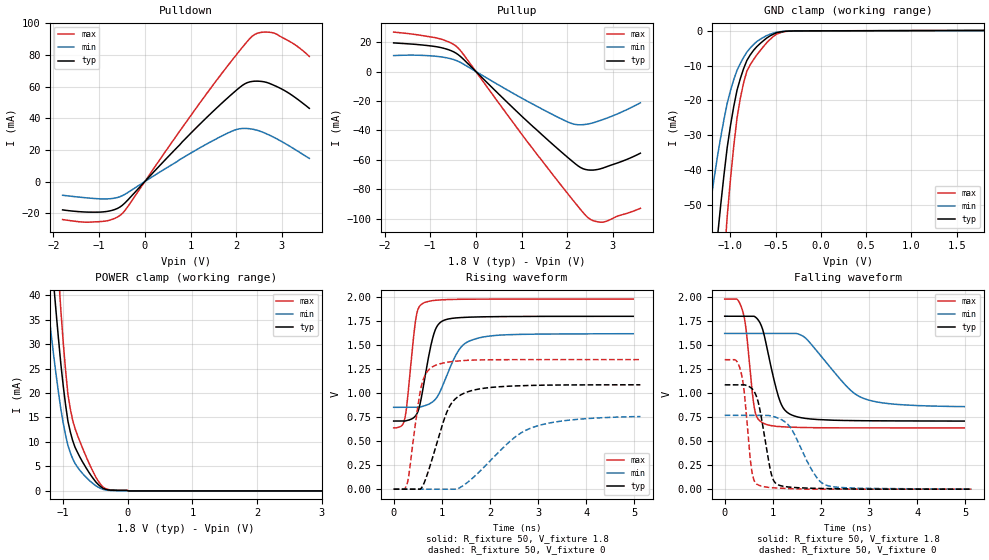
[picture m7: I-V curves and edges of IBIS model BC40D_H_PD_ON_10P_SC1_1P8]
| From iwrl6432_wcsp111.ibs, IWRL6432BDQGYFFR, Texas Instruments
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|   Model Cell BC40D_H_PD_ON_10P_SC1_1P8
|BC40D_H_PD_ON_10P_SC1_1P8
[Model]   BC40D_H_PD_ON_10P_SC1_1P8
Model_type   I/O
Polarity   Non-Inverting
Enable   Active-Low
Vinl =  0.63
Vinh =  1.17
Cref =  15pF
Rref =  100.0000M
Vref =  0V
Vmeas =  0.9
C_comp   2.389419p   2.292106p   2.408415p
|[Input load] weak_pd_on
|[Output drive] slow
|[supplytol] 10
|[temp] ind
[Model Spec]
Vinl   0.63   0.567   0.693
Vinh   1.17   1.053   1.287
[Temperature Range]   25   125   -40
[Voltage Range]   1.8   1.62   1.98
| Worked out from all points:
|   slope of the pulldown table from 0 to 0.27 V, typ, clamps not added: 32.2 ohm
|   slope of the pullup table from 0 to 0.27 V, typ, clamps not added: 32.6 ohm
|   GND clamp passes 1 mA (typ) near -0.53 V on its own axis
|   POWER clamp passes 1 mA (typ) near -0.43 V on its own axis
|   rising waveform, R_fixture 50, V_fixture 1.8: 20-80 % time 249ps typ, 424ps min, 162ps max; typ from 0.709 V to 1.8 V
|   rising waveform, R_fixture 50, V_fixture 0: 20-80 % time 429ps typ, 994ps min, 231ps max; typ from 0 V to 1.09 V
|   falling waveform, R_fixture 50, V_fixture 1.8: 20-80 % time 310ps typ, 792ps min, 166ps max; typ from 1.8 V to 0.708 V
|   falling waveform, R_fixture 50, V_fixture 0: 20-80 % time 227ps typ, 467ps min, 151ps max; typ from 1.08 V to 0 V
| Nom Voltages:
|   VDD=1.1001, VDDS=1.8, VDDS18=1.8, ESD_BIASFET=0, VSS=0, VSSS=0
| Min Voltages:
|   VDD=0.99, VDDS=1.62, VDDS18=1.62, ESD_BIASFET=0, VSS=0, VSSS=0
| Max Voltages:
|   VDD=1.21, VDDS=1.98, VDDS18=1.98, ESD_BIASFET=0, VSS=0, VSSS=0
[POWER_clamp]
|   voltage   I(typ)   I(min)   I(max)
-1.8V     158.9mA    112.6mA    219.9mA
-1.255V   60.04mA    40.04mA    85.04mA
-1.145V   41.99mA    27.45mA    59.9mA
-1.109V   36.4mA     23.66mA    51.96mA
-1.073V   31.03mA    20.08mA    44.3mA
-1.036V   25.91mA    16.71mA    36.9mA
-927.3mV  14.27mA    9.297mA    19.77mA
-854.5mV  10.33mA    6.619mA    14.49mA
-454.5mV  1.273mA    741.7uA    1.94mA
-309.1mV  221.6uA    132.8uA    307.9uA
18.18mV   0A         0A         0A
3.6V      0A         0A         0A
[Pulldown]
|   voltage   I(typ)   I(min)   I(max)
-1.8V     -17.92mA   -8.674mA   -24.03mA
-927.3mV  -19.22mA   -10.99mA   -25.2mA
-654.5mV  -17.65mA   -10.46mA   -23.22mA
-490.9mV  -14.97mA   -8.904mA   -20.12mA
818.2mV   25.05mA    14.78mA    34.16mA
1.691V    49.7mA     28.87mA    68.58mA
2.127V    60.63mA    33.53mA    84.59mA
2.4V      63.43mA    32.85mA    92.9mA
2.618V    62.99mA    30.74mA    94.47mA
2.836V    60.69mA    27.76mA    93.76mA
3.273V    53.49mA    20.53mA    86.73mA
3.6V      46.26mA    14.64mA    79.12mA
[Pullup]
|   voltage   I(typ)   I(min)   I(max)
-1.8V     19.42mA    10.82mA    26.76mA
-818.2mV  16.58mA    10.15mA    22.47mA
-545.5mV  14.19mA    8.648mA    19.37mA
-381.8mV  11.34mA    6.842mA    15.75mA
1.036V    -31.26mA   -18.6mA    -43.9mA
1.909V    -55.59mA   -32.73mA   -78.89mA
2.182V    -62.71mA   -35.92mA   -89.46mA
2.345V    -65.94mA   -36.05mA   -95.62mA
2.455V    -66.75mA   -35.58mA   -99.18mA
2.618V    -66.67mA   -34.29mA   -101.7mA
2.782V    -65.46mA   -32.56mA   -102.2mA
3.6V      -55.4mA    -21.22mA   -92.82mA
[GND_clamp]
|   voltage   I(typ)   I(min)   I(max)
-1.8V     -270.2mA   -170.2mA   -430.1mA
-1.255V   -91.66mA   -55.91mA   -148.4mA
-1.145V   -59.91mA   -36.45mA   -97.1mA
-1.109V   -50.48mA   -30.83mA   -81.56mA
-1.073V   -41.73mA   -25.65mA   -67.06mA
-1.036V   -33.67mA   -20.93mA   -53.6mA
-927.3mV  -17.08mA   -11.35mA   -25.06mA
-854.5mV  -10.88mA   -7.623mA   -14.95mA
-781.8mV  -6.944mA   -4.955mA   -9.81mA
-636.4mV  -2.852mA   -1.883mA   -4.568mA
-381.8mV  -107.5uA   -91.83uA   -158.4uA
1.8V      101.9uA    59.86uA    152.6uA
[Ramp]
| variable   typ   min   max
dV/dt_f  0.6608501/0.31247664n 0.46735341/0.81405775n 0.80986843/0.1677152n
dV/dt_r 0.65873657/0.43263011n 0.47402485/1.0517225n 0.81471545/0.23230577n
R_load = 50
[Rising Waveform]
R_fixture = 50
V_fixture = 1.8
V_fixture_min = 1.62
V_fixture_max = 1.98
|   time   V(typ)   V(min)   V(max)
0s        708.5mV    851.3mV    637.8mV
228.1ps   708.5mV    851.3mV    726mV
278.6ps   714.1mV    851.3mV    895.7mV
459.6ps   765.9mV    851.6mV    1.77V
612.3ps   1.054V     862.9mV    1.934V
841.8ps   1.626V     922.1mV    1.963V
1.074ns   1.762V     1.145V     1.971V
1.389ns   1.785V     1.471V     1.975V
1.777ns   1.792V     1.574V     1.977V
4.974ns   1.798V     1.617V     1.977V
[Rising Waveform]
R_fixture = 50
V_fixture = 0
V_fixture_min = 0
V_fixture_max = 0
|   time   V(typ)   V(min)   V(max)
0s        0V         0V         0V
273.6ps   0V         0V         47.5mV
570.6ps   8.425mV    0V         1.06V
671ps     114mV      0V         1.202V
834.9ps   374.1mV    0V         1.28V
1.166ns   866mV      0V         1.324V
1.554ns   1.016V     78.57mV    1.341V
2.437ns   1.072V     507.4mV    1.347V
2.86ns    1.079V     637.3mV    1.347V
5.123ns   1.086V     754.9mV    1.348V
[Falling Waveform]
R_fixture = 50
V_fixture = 1.8
V_fixture_min = 1.62
V_fixture_max = 1.98
|   time   V(typ)   V(min)   V(max)
0s        1.799V     1.619V     1.977V
369ps     1.799V     1.619V     1.859V
442.1ps   1.799V     1.619V     1.669V
618.1ps   1.796V     1.619V     837.9mV
787.7ps   1.662V     1.619V     689.6mV
1.129ns   942.3mV    1.619V     651.2mV
1.383ns   773.4mV    1.619V     644.4mV
1.679ns   735.8mV    1.571V     640.6mV
2.85ns    711.8mV    951.1mV    637.2mV
4.974ns   708.1mV    858.7mV    637mV
[Falling Waveform]
R_fixture = 50
V_fixture = 0
V_fixture_min = 0
V_fixture_max = 0
|   time   V(typ)   V(min)   V(max)
0s        1.085V     768mV      1.347V
329.5ps   1.085V     768mV      1.235V
404.9ps   1.085V     768mV      1.014V
556.5ps   1.05V      768mV      209.1mV
687.9ps   920.5mV    768mV      45.88mV
960ps     173.5mV    761.9mV    15.98mV
1.117ns   43.4mV     737.3mV    11.07mV
1.37ns    20.15mV    638.2mV    4.644mV
2.109ns   5.655mV    41.02mV    0V
5.123ns   0V         0V         0V
